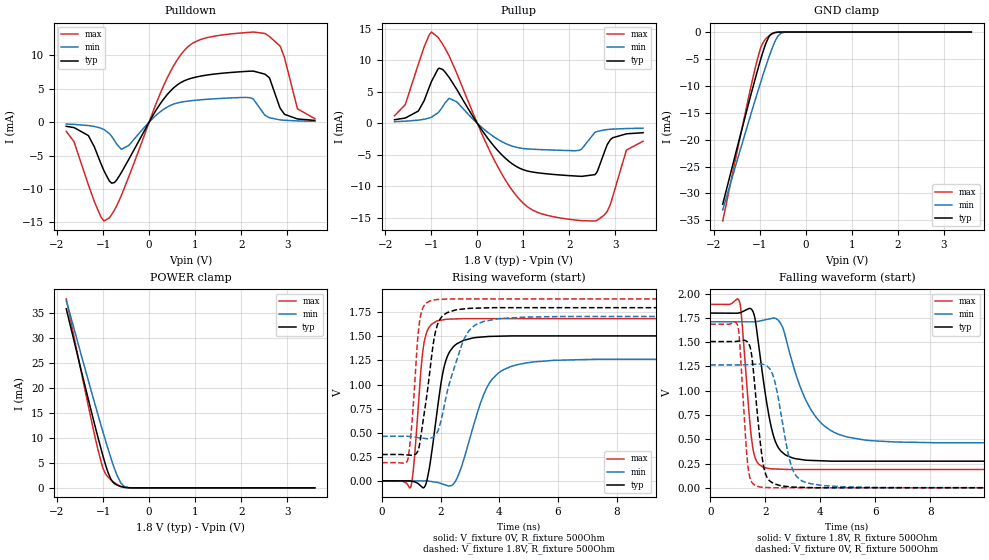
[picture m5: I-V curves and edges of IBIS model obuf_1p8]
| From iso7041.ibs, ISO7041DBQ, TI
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|   obuf_1p8 Model
[Model]   obuf_1p8
Model_type   3-state
Polarity   Non-Inverting
Vmeas = 0.9
Vref = 0
Cref = 2pF
Rref = 100000
|   typ   min   max
C_comp   0.494pF   0.461pF   0.567pF
| Where Nom  PVT is Nominal Process, 1.8V, 27C
|   Fast PVT is Strong Process,  1.89V, -55C
|   Slow PVT is Weak Process,   1.71V, 150C
[Voltage Range]   1.8   1.71   1.89
|Junction Temperature
[Temperature Range]   27   150   -55
[Pullup Reference]   1.8   1.71   1.89
[Pulldown Reference]   0   0   0
[Power Clamp Reference]   1.8   1.71   1.89
[GND Clamp Reference]   0   0   0
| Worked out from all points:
|   slope of the pulldown table from 0 to 0.27 V, typ, clamps not added: 89.4 ohm
|   slope of the pullup table from 0 to 0.27 V, typ, clamps not added: 96.7 ohm
|   GND clamp passes 1 mA (typ) near -0.80 V on its own axis
|   POWER clamp passes 1 mA (typ) near -0.77 V on its own axis
|   falling waveform, V_fixture 1.8V, R_fixture 500Ohm: 20-80 % time 510ps typ, 1.07ns min, 295ps max; typ from 1.8 V to 0.273 V
|   rising waveform, V_fixture 0V, R_fixture 500Ohm: 20-80 % time 438ps typ, 838ps min, 261ps max; typ from 0 V to 1.51 V
|   rising waveform, V_fixture 1.8V, R_fixture 500Ohm: 20-80 % time 409ps typ, 707ps min, 240ps max; typ from 0.273 V to 1.8 V
|   falling waveform, V_fixture 0V, R_fixture 500Ohm: 20-80 % time 325ps typ, 508ps min, 228ps max; typ from 1.51 V to 0 V
[Pulldown]
|   Voltage   I(typ)   I(min)   I(max)
-1.8V     -623.6uA   -287.2uA   -1.385mA
-1.319V   -2.01mA    -512.9uA   -9.376mA
-979.2mV  -7.295mA   -1.112mA   -14.79mA
-811.8mV  -9.129mA   -2.137mA   -13.81mA
-606.6mV  -7.59mA    -4.065mA   -11.04mA
387mV     4.069mA    2.224mA    6.509mA
991.8mV   6.695mA    3.26mA     11.97mA
2.201V    7.621mA    3.632mA    13.44mA
2.515V    7.175mA    1.035mA    13.26mA
2.936V    1.213mA    280.7uA    9.749mA
3.222V    474.5uA    182.2uA    1.988mA
3.6V      257.7uA    123.7uA    521.7uA
[GND Clamp]
|   Voltage   I(typ)   I(min)   I(max)
-1.8V     -32mA      -33.06mA   -35.12mA
-1.454V   -20.4mA    -22.93mA   -20.84mA
-1.076V   -8.127mA   -12.12mA   -6.028mA
-990mV    -5.506mA   -9.735mA   -3.3mA
-941.4mV  -4.112mA   -8.417mA   -2.233mA
-860.4mV  -2.045mA   -6.278mA   -1.213mA
-801mV    -932.3uA   -4.776mA   -740.9uA
-736.2mV  -316.1uA   -3.239mA   -383uA
-606.6mV  -29.73uA   -830.3uA   -42.38uA
-536.4mV  -6.709uA   -216.1uA   -7.734uA
-444.6mV  -752.4nA   -22.17uA   -540.1nA
3.6V      0A         0A         0A
[Pullup]
|   Voltage   I(typ)   I(min)   I(max)
-1.8V     581.6uA    270.4uA    1.218mA
-1.568V   851.3uA    343.8uA    2.963mA
-1.282V   1.96mA     515.4uA    9.414mA
-995.4mV  6.681mA    996.1uA    14.53mA
-612mV    7.306mA    3.994mA    10.72mA
462.6mV   -4.473mA   -2.616mA   -7.146mA
1.219V    -7.761mA   -4.117mA   -13.85mA
2.207V    -8.401mA   -4.289mA   -15.43mA
2.606V    -7.64mA    -1.281mA   -15.39mA
2.936V    -2.297mA   -913.2uA   -11.76mA
3.238V    -1.659mA   -817.8uA   -4.238mA
3.6V      -1.484mA   -766.6uA   -2.84mA
[POWER Clamp]
|   Voltage   I(typ)   I(min)   I(max)
-1.8V     35.76mA    37.47mA    37.75mA
-1.438V   22.06mA    25.32mA    21.52mA
-1.103V   9.809mA    14.35mA    7.297mA
-1.012V   6.671mA    11.44mA    4.168mA
-952.2mV  4.775mA    9.594mA    2.895mA
-887.4mV  2.947mA    7.633mA    2.113mA
-784.8mV  1.124mA    4.7mA      1.237mA
-698.4mV  561.1uA    2.534mA    681.4uA
-612mV    251.5uA    947.6uA    275.5uA
-547.2mV  108.1uA    334.3uA    95.72uA
-444.6mV  15.08uA    50.06uA    7.661uA
3.6V      0A         0A         0A
[Ramp]
R_load = 500
|   typ   min   max
dV/dt_r   0.903987/4.37721e-10   0.759811/8.37625e-10   1.01141/2.60297e-10
dV/dt_f   0.915973/5.08971e-10   0.748503/1.07333e-09   1.02088/2.94484e-10
[Falling Waveform]
V_fixture = 1.8V
V_fixture_min = 1.71V
V_fixture_max = 1.89V
R_fixture = 500Ohm
C_fixture = 0F
|   Time   V(typ)   V(min)   V(max)
0s        1.8V       1.71V      1.89V
1.049ns   1.802V     1.71V      1.927V
1.115ns   1.807V     1.709V     1.825V
1.573ns   1.801V     1.709V     372.8mV
2.192ns   661mV      1.743V     196.2mV
2.705ns   345.1mV    1.589V     190.5mV
3.328ns   291mV      999.9mV    189.3mV
4.057ns   278.4mV    661.7mV    189.3mV
6.723ns   274.7mV    472.2mV    189.3mV
150ns     273.4mV    462.5mV    188.5mV
[Rising Waveform]
V_fixture = 0V
V_fixture_min = 0V
V_fixture_max = 0V
R_fixture = 500Ohm
C_fixture = 0F
|   Time   V(typ)   V(min)   V(max)
0s        -832.8nV   -130.1nV   -8.35nV
988.2ps   -2.038mV   -608uV     -52.35mV
1.103ns   -9.767mV   -678.9uV   235.8mV
1.354ns   -61.97mV   -833.2uV   1.249V
1.469ns   -53.16mV   -903.5uV   1.487V
2.192ns   1.264V     -46.63mV   1.678V
2.569ns   1.427V     35.38mV    1.682V
3.747ns   1.501V     1.054V     1.685V
5.864ns   1.505V     1.252V     1.685V
150ns     1.507V     1.266V     1.686V
[Rising Waveform]
V_fixture = 1.8V
V_fixture_min = 1.71V
V_fixture_max = 1.89V
R_fixture = 500Ohm
C_fixture = 0F
|   Time   V(typ)   V(min)   V(max)
0s        273.4mV    462.5mV    188.5mV
881.1ps   268.3mV    462.5mV    225.8mV
1.025ns   264.9mV    457mV      622.7mV
1.218ns   307.8mV    449.6mV    1.482V
1.404ns   633.6mV    442.5mV    1.804V
1.909ns   1.637V     522.3mV    1.884V
2.325ns   1.757V     1.043V     1.889V
2.973ns   1.791V     1.561V     1.889V
4.811ns   1.799V     1.7V       1.889V
150ns     1.8V       1.71V      1.89V
[Falling Waveform]
|Gnd
V_fixture = 0V
V_fixture_min = 0V
V_fixture_max = 0V
R_fixture = 500Ohm
C_fixture = 0F
|   Time   V(typ)   V(min)   V(max)
0s        1.507V     1.266V     1.686V
1.014ns   1.511V     1.266V     1.653V
1.307ns   1.512V     1.268V     425.8mV
1.427ns   1.468V     1.27V      123mV
1.935ns   230.7mV    1.271V     5.087mV
2.284ns   48.9mV     1.156V     599.6uV
2.816ns   13.1mV     374.6mV    598.9uV
3.078ns   7.386mV    142.5mV    598.6uV
4.811ns   1.391mV    11.12mV    596.5uV
150ns     -677.8nV   -554.7nV   -8.151nV
